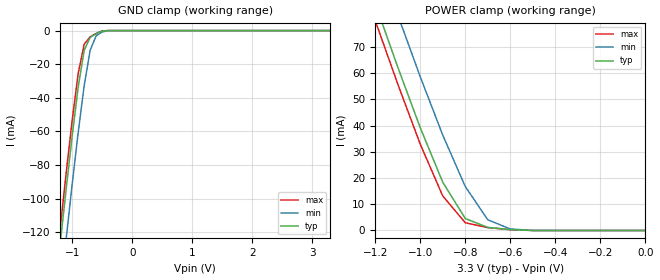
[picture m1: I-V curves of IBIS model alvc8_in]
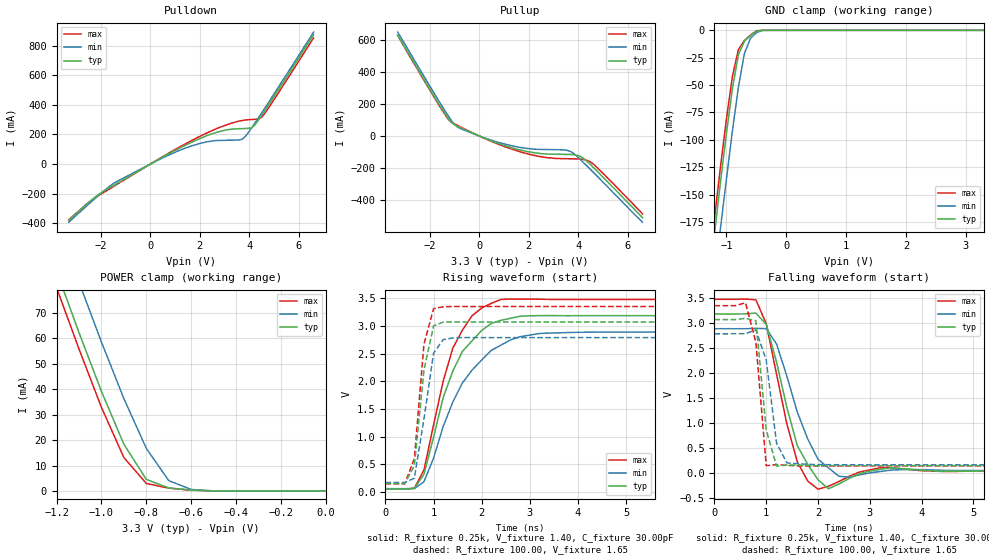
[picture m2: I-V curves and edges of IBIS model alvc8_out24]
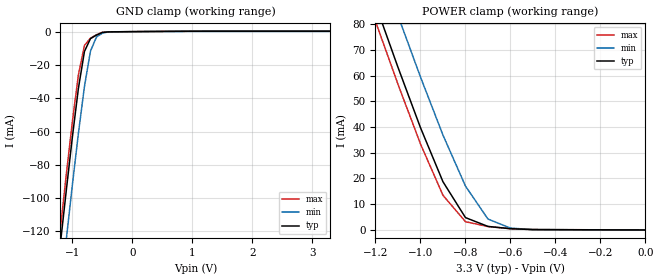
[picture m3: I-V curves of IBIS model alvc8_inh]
| IBIS file 32244ah.ibs created by s2ibis2 version 1.1
| North Carolina State University Electronics Research Laboratory  1995
[IBIS ver]   2.1
[File name]   32244ah.ibs
[File Rev]   1.0
[Date]   03/01/99
[Source]   Integrated Device Technology, Inc.
[Notes]   1.Temperatures: typ=25C, min=100C, max=0C 2.RRmp rates based
   on 50 ohm load.
[Disclaimer] Integrated Device Technology, Inc. ("IDT") hereby grants the
   user of this IBIS model a non-exclusive, nontransferable
   license to use this IBIS model under the following terms. The
   user is granted this license only to use the IBIS model and is
   not granted rights to sell, copy (except as needed to run the
   IBIS model), rent, lease or sub-license the IBIS model in
   whole or in part, or in modified form to anyone. The User may
   modify the IBIS model to suit its specific applications, but
   rights to derivative works and such modifications shall belong
   to IDT. This IBIS model is provided on an AS IS" basis and IDT
   makes absolutely no warranty with respect to the information
   contained herein. IDT DISCLAIMS AND CUSTOMER WAIVES ALL
   WARRANTIES, EXPRESS AND IMPLIED, INCLUDING WARRANTIES OF
   MERCHANTABILITY AND FITNESS FOR A PARTICULAR PURPOSE. THE
   ENTIRE RISK AS TO QUALITY AND PERFORMANCE IS WITH THE USER
   ACCORDINGLY, IN NO EVENT SHALL IDT BE LIABLE FOR ANY DIRECT OR
   INDIRECT DAMAGES, WHETHER IN CONTRACT OR TORT, INCLUDING ANY
   LOST PROFITS OR OTHER INCIDENTAL, CONSEQUENTIAL, EXEMPLARY, OR
   PUNITIVE DAMAGES ARISING OUT OF THE USE OR APPLICATION OF THE
   IBIS model. Further, IDT reserves the right to make changes
   without notice to any product herein to improve reliability,
   function, or design. IDT does not convey any license under
   patent rights or any other intellectual property rights,
   including those of third parties. IDT is not obligated to
   provide maintenance or support for the licensed IBIS model.
[Copyright]   Copyright 1997, Integrated Device Technology, Inc. all rights
   reserved
|   Component ALVCH32244
[Component]   ALVCH32244
[Manufacturer]   Integrated Device Technology
[Package]
| BF96
| variable   typ   min   max
R_pkg   144.3m   NA   NA
L_pkg   4.10nH   NA   NA
C_pkg   0.36pF   NA   NA
[Pin]  signal_name   model_name   R_pin   L_pin   C_pin
A1   1Y2   alvc8_out24
A2   1Y1   alvc8_out24
A3   1OEB   alvc8_in
A4   2OEB   alvc8_in
A5   1A1   alvc8_inh
A6   1A2   alvc8_inh
B1   1Y4   alvc8_out24
B2   1Y3   alvc8_out24
B3   GND   GND
B4   GND   GND
B5   1A3   alvc8_inh
B6   1A4   alvc8_inh
C1   2Y2   alvc8_out24
C2   2Y1   alvc8_out24
C3   VCC   POWER
C4   VCC   POWER
C5   2A1   alvc8_inh
C6   2A2   alvc8_inh
D1   2Y4   alvc8_out24
D2   2Y3   alvc8_out24
D3   GND   GND
D4   GND   GND
D5   2A3   alvc8_inh
D6   2A4   alvc8_inh
E1   3Y2   alvc8_out24
E2   3Y1   alvc8_out24
E3   GND   GND
E4   GND   GND
E5   3A1   alvc8_out24
E6   3A2   alvc8_out24
F1   3Y4   alvc8_out24
F2   3Y3   alvc8_out24
F3   VCC   POWER
F4   VCC   POWER
F5   3A3   alvc8_inh
F6   3A4   alvc8_inh
G1   4Y2   alvc8_out24
G2   4Y1   alvc8_out24
G3   GND   GND
G4   GND   GND
G5   4A1   alvc8_inh
G6   4A2   alvc8_inh
H1   4Y3   alvc8_out24
H2   4Y4   alvc8_out24
H3   4OEB   alvc8_in
H4   3OEB   alvc8_in
H5   4A4   alvc8_inh
H6   4A3   alvc8_inh
J1   5Y2   alvc8_out24
J2   5Y1   alvc8_out24
J3   5OEB   alvc8_in
J4   6OEB   alvc8_in
J5   5A1   alvc8_inh
J6   5A2   alvc8_inh
K1   5Y4   alvc8_out24
K2   5Y3   alvc8_out24
K3   GND   GND
K4   GND   GND
K5   5A3   alvc8_inh
K6   5A4   alvc8_inh
L1   6Y2   alvc8_out24
L2   6Y1   alvc8_out24
L3   VCC   POWER
L4   VCC   POWER
L5   6A1   alvc8_inh
L6   6A2   alvc8_inh
M1   6Y4   alvc8_out24
M2   6Y3   alvc8_out24
M3   GND   GND
M4   GND   GND
M5   6A3   alvc8_inh
M6   6A4   alvc8_inh
N1   7Y2   alvc8_out24
N2   7Y1   alvc8_out24
N3   GND   GND
N4   GND   GND
N5   7A1   alvc8_out24
N6   7A2   alvc8_out24
P1   7Y4   alvc8_out24
P2   7Y3   alvc8_out24
P3   VCC   POWER
P4   VCC   POWER
P5   7A3   alvc8_inh
P6   7A4   alvc8_inh
R1   8Y2   alvc8_out24
R2   8Y1   alvc8_out24
R3   GND   GND
R4   GND   GND
R5   8A1   alvc8_inh
R6   8A2   alvc8_inh
T1   8Y3   alvc8_out24
T2   8Y4   alvc8_out24
T3   8OEB   alvc8_in
T4   7OEB   alvc8_in
T5   8A4   alvc8_inh
T6   8A3   alvc8_inh
| Models and submodels in the file (3): alvc8_in (Input), alvc8_out24 (3-state), alvc8_inh (Input)
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| in   in   dummy_model
| oe   oe   dummy_model
|   Model alvc8_in
[Model]   alvc8_in
Model_type   Input
Vinl =  0.800V
Vinh =  2.000V
C_comp   3.00pF   NA   NA
[Temperature Range]   25.00   100.00   0.000
[Voltage Range]   3.30V   3.00V   3.60V
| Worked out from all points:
|   GND clamp passes 1 mA (typ) near -0.54 V on its own axis
|   POWER clamp passes 1 mA (typ) near -0.68 V on its own axis
[GND_clamp]
| voltage   I(typ)   I(min)   I(max)
-3.3V     -860mA     -887mA     -851mA
-1.3V     -161mA     -190mA     -151mA
-1.2V     -127mA     -157mA     -118mA
-1.1V     -94.41mA   -124mA     -84.85mA
-1V       -62.78mA   -91.54mA   -53.52mA
-900mV    -33.71mA   -60.78mA   -25.6mA
-800mV    -11.74mA   -32.83mA   -8.09mA
-700mV    -4.033mA   -11.65mA   -3.7mA
-600mV    -1.899mA   -3.108mA   -1.699mA
-500mV    -308uA     -810uA     -172uA
-400mV    -3.848nA   -9.872uA   -399pA
3.3V      39.6pA     19.33nA    26.4pA
[POWER_clamp]
| voltage   I(typ)   I(min)   I(max)
-3.3V     630mA      648mA      624mA
-1.2V     86.56mA    106mA      80.02mA
-1.1V     62.33mA    82.22mA    55.88mA
-1V       39.2mA     58.61mA    32.91mA
-900mV    18.4mA     36.35mA    13.15mA
-800mV    4.556mA    16.76mA    2.954mA
-700mV    1.164mA    4.056mA    1.087mA
-600mV    320uA      578uA      299uA
-500mV    40.08nA    12.23uA    3.465nA
0V        39.6pA     59.11pA    43.2pA
|   Model alvc8_out24
[Model]   alvc8_out24
Model_type   3-state
Polarity   Non-Inverting
Enable   Active-High
Vmeas =  1.500V
C_comp   3.00pF   NA   NA
[Temperature Range]   25.00   100.00   0.000
[Voltage Range]   3.30V   3.00V   3.60V
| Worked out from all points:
|   slope of the pulldown table from 0 to 0.495 V, typ, clamps not added: 10.5 ohm
|   slope of the pullup table from 0 to 0.495 V, typ, clamps not added: 16.1 ohm
|   GND clamp passes 1 mA (typ) near -0.50 V on its own axis
|   POWER clamp passes 1 mA (typ) near -0.68 V on its own axis
|   rising waveform, R_fixture 0.25k, V_fixture 1.40, C_fixture 30.00pF: 20-80 % time 712ps typ, 930ps min, 636ps max; typ from 0.056 V to 3.19 V
|   rising waveform, R_fixture 100.00, V_fixture 1.65: 20-80 % time 241ps typ, 276ps min, 194ps max; typ from 0.155 V to 3.08 V
|   falling waveform, R_fixture 0.25k, V_fixture 1.40, C_fixture 30.00pF: 20-80 % time 456ps typ, 551ps min, 426ps max; typ from 3.19 V to 0.056 V
|   falling waveform, R_fixture 100.00, V_fixture 1.65: 20-80 % time 185ps typ, 189ps min, 171ps max; typ from 3.08 V to 0.155 V
[Pulldown]
| voltage   I(typ)   I(min)   I(max)
-3.3V     -381mA     -393mA     -377mA
-2.2V     -219mA     -227mA     -224mA
-1.5V     -146mA     -132mA     -153mA
500mV     47.5mA     41.7mA     49.9mA
1.4V      126mA      107mA      135mA
2.3V      193mA      151mA      211mA
3.1V      232mA      161mA      266mA
3.7V      239mA      167mA      294mA
4.1V      246mA      246mA      301mA
4.5V      329mA      345mA      316mA
5.1V      483mA      500mA      461mA
6.6V      875mA      892mA      853mA
[Pullup]
| voltage   I(typ)   I(min)   I(max)
-3.3V     630mA      649mA      628mA
-1.4V     142mA      160mA      137mA
-1.1V     80.6mA     90.7mA     83.6mA
-900mV    63mA       57.7mA     67.6mA
400mV     -25.1mA    -21.5mA    -27.4mA
1.6V      -85mA      -69.5mA    -95.9mA
2.6V      -111mA     -84mA      -132mA
3.4V      -115mA     -86.1mA    -141mA
3.7V      -115mA     -97.1mA    -142mA
4.1V      -128mA     -149mA     -144mA
4.5V      -179mA     -210mA     -162mA
6.6V      -510mA     -538mA     -486mA
[GND_clamp]
| voltage   I(typ)   I(min)   I(max)
-3.3V     -1.227A    -1.266A    -1.214A
-1.3V     -233mA     -276mA     -219mA
-1.2V     -186mA     -228mA     -172mA
-1.1V     -139mA     -181mA     -125mA
-1V       -94.27mA   -136mA     -81.1mA
-900mV    -53.23mA   -91.93mA   -42.09mA
-800mV    -22.31mA   -52.04mA   -17.61mA
-700mV    -9.958mA   -21.29mA   -9.325mA
-600mV    -4.943mA   -7.436mA   -4.424mA
-500mV    -830uA     -2.115mA   -472uA
-400mV    -8.73nA    -25.66uA   -695pA
3.3V      92.41pA    19.42nA    79.2pA
[POWER_clamp]
| voltage   I(typ)   I(min)   I(max)
-3.3V     630mA      648mA      624mA
-1.2V     86.56mA    106mA      80.02mA
-1.1V     62.33mA    82.22mA    55.88mA
-1V       39.2mA     58.61mA    32.91mA
-900mV    18.4mA     36.35mA    13.15mA
-800mV    4.556mA    16.76mA    2.954mA
-700mV    1.164mA    4.056mA    1.087mA
-600mV    320uA      578uA      299uA
-500mV    40.14nA    12.23uA    3.53nA
0V        92.41pA    138pA      101pA
[Ramp]
| variable   typ   min   max
dV/dt_r   1.48/0.31n   1.29/0.30n   1.66/0.22n
dV/dt_f   1.63/0.28n   1.45/0.31n   1.80/0.19n
R_load = 50.00
[Rising Waveform]
R_fixture = 0.25k
V_fixture = 1.40
C_fixture = 30.00pF
R_dut = 144.30m
L_dut = 4.10nH
C_dut = 0.36pF
| time   V(typ)   V(min)   V(max)
0s        55.61mV    62.15mV    53.22mV
600ps     67.1mV     63.76mV    71.36mV
800ps     323mV      188mV      399mV
1.2ns     1.71V      1.187V     2.006V
1.4ns     2.186V     1.627V     2.602V
1.8ns     2.733V     2.205V     3.187V
2.4ns     3.104V     2.656V     3.482V
2.8ns     3.179V     2.809V     3.489V
4ns       3.189V     2.888V     3.48V
19.8ns    3.189V     2.893V     3.481V
[Rising Waveform]
R_fixture = 100.00
V_fixture = 1.65
R_dut = 144.30m
L_dut = 4.10nH
C_dut = 0.36pF
| time   V(typ)   V(min)   V(max)
0s        155mV      173mV      149mV
400ps     155mV      173mV      149mV
600ps     476mV      252mV      604mV
800ps     2.207V     1.324V     2.674V
1ns       3.005V     2.511V     3.315V
1.2ns     3.072V     2.757V     3.349V
1.4ns     3.076V     2.786V     3.355V
1.6ns     3.076V     2.793V     3.354V
19.8ns    3.076V     2.792V     3.354V
[Falling Waveform]
R_fixture = 0.25k
V_fixture = 1.40
C_fixture = 30.00pF
R_dut = 144.30m
L_dut = 4.10nH
C_dut = 0.36pF
| time   V(typ)   V(min)   V(max)
0s        3.189V     2.893V     3.481V
800ps     3.206V     2.901V     3.471V
1ns       2.981V     2.895V     2.993V
1.2ns     2.223V     2.586V     1.98V
1.6ns     557mV      1.227V     234mV
2ns       -126mV     283mV      -314mV
2.2ns     -306mV     114mV      -257mV
2.4ns     -213mV     -54.48mV   -163mV
3.2ns     82.67mV    38.85mV    114mV
19.8ns    55.61mV    62.15mV    53.23mV
[Falling Waveform]
R_fixture = 100.00
V_fixture = 1.65
R_dut = 144.30m
L_dut = 4.10nH
C_dut = 0.36pF
| time   V(typ)   V(min)   V(max)
0s        3.076V     2.792V     3.354V
400ps     3.076V     2.793V     3.354V
600ps     3.101V     2.794V     3.411V
800ps     3.052V     2.869V     2.626V
1ns       869mV      2.268V     155mV
1.2ns     147mV      602mV      178mV
1.4ns     168mV      211mV      161mV
2ns       153mV      177mV      149mV
2.8ns     155mV      173mV      149mV
19.8ns    155mV      173mV      149mV
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|   Model alvc8_inh
[Model]   alvc8_inh
Model_type   Input
Vinl =  0.800V
Vinh =  2.000V
C_comp   3.00pF   NA   NA
[Temperature Range]   25.00   100.00   0.000
[Voltage Range]   3.30V   3.00V   3.60V
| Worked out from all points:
|   GND clamp passes 1 mA (typ) near -0.53 V on its own axis
|   POWER clamp passes 1 mA (typ) near -0.66 V on its own axis
[GND_clamp]
| voltage   I(typ)   I(min)   I(max)
-3.3V     -860mA     -888mA     -852mA
-1.3V     -161mA     -190mA     -151mA
-1.2V     -127mA     -157mA     -118mA
-1.1V     -94.51mA   -124mA     -84.99mA
-1V       -62.91mA   -91.62mA   -53.71mA
-900mV    -33.88mA   -60.87mA   -25.82mA
-800mV    -11.92mA   -32.93mA   -8.306mA
-700mV    -4.211mA   -11.77mA   -3.908mA
-600mV    -2.051mA   -3.213mA   -1.882mA
-500mV    -472uA     -914uA     -379uA
-400mV    -144uA     -112uA     -169uA
3.3V      264uA      163uA      349uA
[POWER_clamp]
| voltage   I(typ)   I(min)   I(max)
-3.3V     638mA      656mA      632mA
-1.2V     87.67mA    108mA      81.05mA
-1.1V     63.19mA    83.28mA    56.62mA
-1V       39.75mA    59.43mA    33.41mA
-900mV    18.73mA    36.86mA    13.47mA
-800mV    4.8mA      17.05mA    3.222mA
-700mV    1.374mA    4.243mA    1.32mA
-600mV    498uA      728uA      497uA
-500mV    146uA      134uA      162uA
0V        45.19pA    64.49pA    49.16pA
